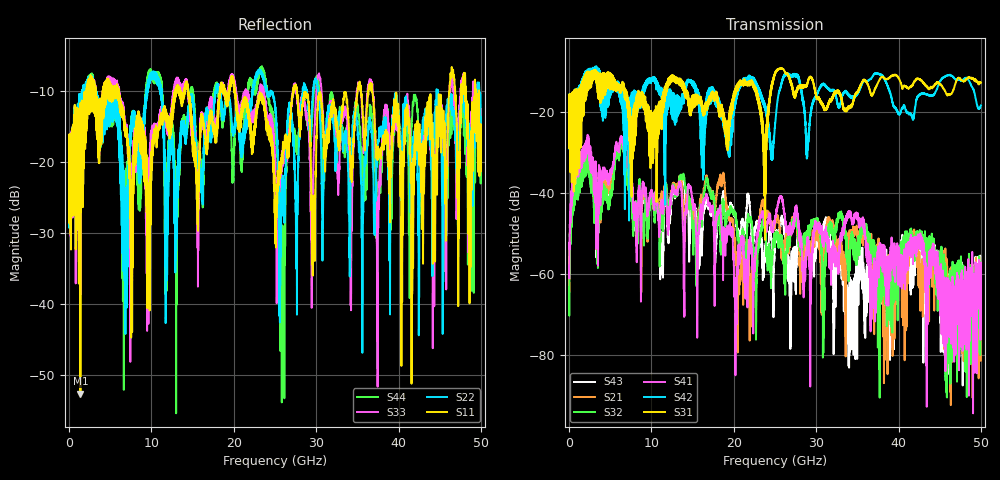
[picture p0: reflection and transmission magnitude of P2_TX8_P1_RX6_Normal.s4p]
!Keysight Technologies,N5225B,MY57041031,A.13.20.10
!Date: Friday, May 31, 2019 11:23:46
!Correction: S11(Full 4 Port(1,2,3,4))
!S12(Full 4 Port(1,2,3,4))
!S13(Full 4 Port(1,2,3,4))
!S14(Full 4 Port(1,2,3,4))
!S21(Full 4 Port(1,2,3,4))
!S22(Full 4 Port(1,2,3,4))
!S23(Full 4 Port(1,2,3,4))
!S24(Full 4 Port(1,2,3,4))
!S31(Full 4 Port(1,2,3,4))
!S32(Full 4 Port(1,2,3,4))
!S33(Full 4 Port(1,2,3,4))
!S34(Full 4 Port(1,2,3,4))
!S41(Full 4 Port(1,2,3,4))
!S42(Full 4 Port(1,2,3,4))
!S43(Full 4 Port(1,2,3,4))
!S44(Full 4 Port(1,2,3,4))
!S4P File: Measurements: <S11,S12,S13,S14>,
!<S21,S22,S23,S24>,
!<S31,S32,S33,S34>,
!<S41,S42,S43,S44>:
# Hz S  dB  R 50.0
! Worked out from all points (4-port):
!   5000 points, 10 MHz to 50 GHz, reference 50 ohm
!   strongest paths, dB at 10 MHz, 12.51 GHz, 25.01 GHz, 37.51 GHz, 50 GHz:
!     S31: -19.4, -11.5, -10.3, -12.8, -12.8
!     S42: -19.2, -15.6, -23.0, -10.7, -18.4
!     S41: -58.1, -39.4, -46.4, -55.7, -62.3
!     S32: -63.4, -40.2, -52.0, -62.8, -69.3
!     S21: -62.4, -39.1, -48.2, -56.4, -81.5
!     S43: -60.1, -40.8, -52.3, -55.0, -63.7
!   lowest |S11| = -52.6 dB at 1.38 GHz (marker M1), VSWR 1.00, Z = 49.9 - j0.195 ohm
!   |S11| at or under -10 dB: 20.17 GHz to 27.18 GHz (7.008 GHz wide, 29.6 % of centre); 27.67 GHz to 35.03 GHz (7.362 GHz wide, 23.5 % of centre); 36.78 GHz to 46.18 GHz (9.399 GHz wide, 22.7 % of centre)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
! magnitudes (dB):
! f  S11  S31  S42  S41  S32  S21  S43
! 10 MHz  -19.5  -19.4  -19.2  -58.1  -63.4  -62.4  -60.1
! 1.38 GHz  -52.6  -28.8  -17.5  -31.0  -33.8  -32.4  -32.7
! 20.23 GHz  -11.5  -14.5  -17.6  -70.5  -45.4  -55.1  -45.8
! 23.77 GHz  -13.0  -36.6  -19.1  -48.2  -49.9  -45.7  -54.2
! 25.69 GHz  -19.9  -9.3  -13.8  -41.0  -50.4  -52.1  -47.6
! 30.06 GHz  -16.5  -16.7  -16.1  -47.5  -46.7  -48.7  -53.0
! 50 GHz  -14.7  -12.8  -18.4  -62.3  -69.3  -81.5  -63.7
